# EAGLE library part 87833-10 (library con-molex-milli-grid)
HEADER
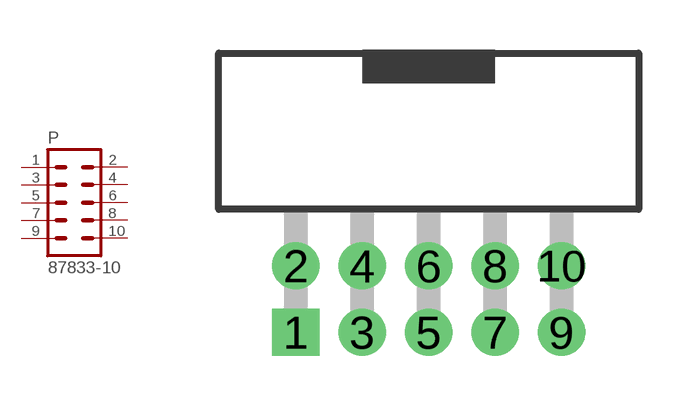
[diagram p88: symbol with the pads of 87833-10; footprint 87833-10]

Designator prefix P

## 87833-10  [87833-10]
1  1  pas
2  2  pas
3  3  pas
4  4  pas
5  5  pas
6  6  pas
7  7  pas
8  8  pas
9  9  pas
10  10  pas

## Footprint 87833-10 (pad centres in mm)
HEADER Dual Row, Shrouded, Right Angle
drill 0.914 square: 1 -4,-1
drill 0.914: 2 -4,1; 3 -2,-1; 4 -2,1; 5 0,-1; 6 0,1; 7 2,-1; 8 2,1; 9 4,-1; 10 4,1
